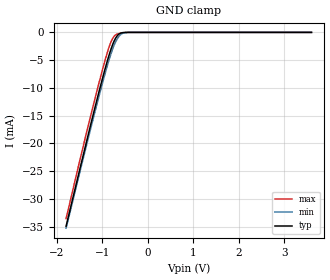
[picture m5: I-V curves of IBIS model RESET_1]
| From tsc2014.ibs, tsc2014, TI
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|   1.8V RESET Model
[Model] RESET_1
Model_type Input
Vinl = 0.54
Vinh = 1.26
|   typ   min   max
C_comp   2.2952570e-12   2.1966560e-12   2.4430410e-12
|Where nom PVT is NOM Process, 1.8V,27C
|   Fast PVT is Strong Process, 2.07V, -40C
|   Slow PVT is Weak Process, 1.53V, 85C
[Model Spec]
Vinl   0.54   0.459   0.621
Vinh   1.26   1.071   1.449
|VINL  0.3 DVDD, VINH  0.7 DVDD
[Voltage Range]   1.8   1.53   2.07
[Temperature Range]   27   85   -40
[Power Clamp Reference]   1.8   1.53   2.07
[GND Clamp Reference]   0   0   0
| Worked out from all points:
|   GND clamp passes 1 mA (typ) near -0.71 V on its own axis
[GND Clamp]
|   Voltage   I(typ)   I(min)   I(max)
-1.8V     -34.91mA   -35.26mA   -33.55mA
-1.338V   -19.27mA   -19.91mA   -17.64mA
-1.089V   -11.1mA    -11.91mA   -9.511mA
-937.8mV  -6.451mA   -7.308mA   -4.884mA
-835mV    -3.601mA   -4.433mA   -2.183mA
-775.4mV  -2.199mA   -2.973mA   -1.1mA
-705.4mV  -976.3uA   -1.622mA   -429.4uA
-638.6mV  -312.1uA   -750.8uA   -225.4uA
-553.2mV  -53uA      -148uA     -85.75uA
-409.7mV  -2.758uA   -2.697uA   -3.248uA
3.6V      0A         0A         0A
[POWER Clamp]
|   SCR cell used for ESD function. Effects occurr above VDD x 2
|   Voltage   I(typ)   I(min)   I(max)
-1.8V     0A         0A         0A
0V        0A         0A         0A
3.6V      0A         0A         0A
